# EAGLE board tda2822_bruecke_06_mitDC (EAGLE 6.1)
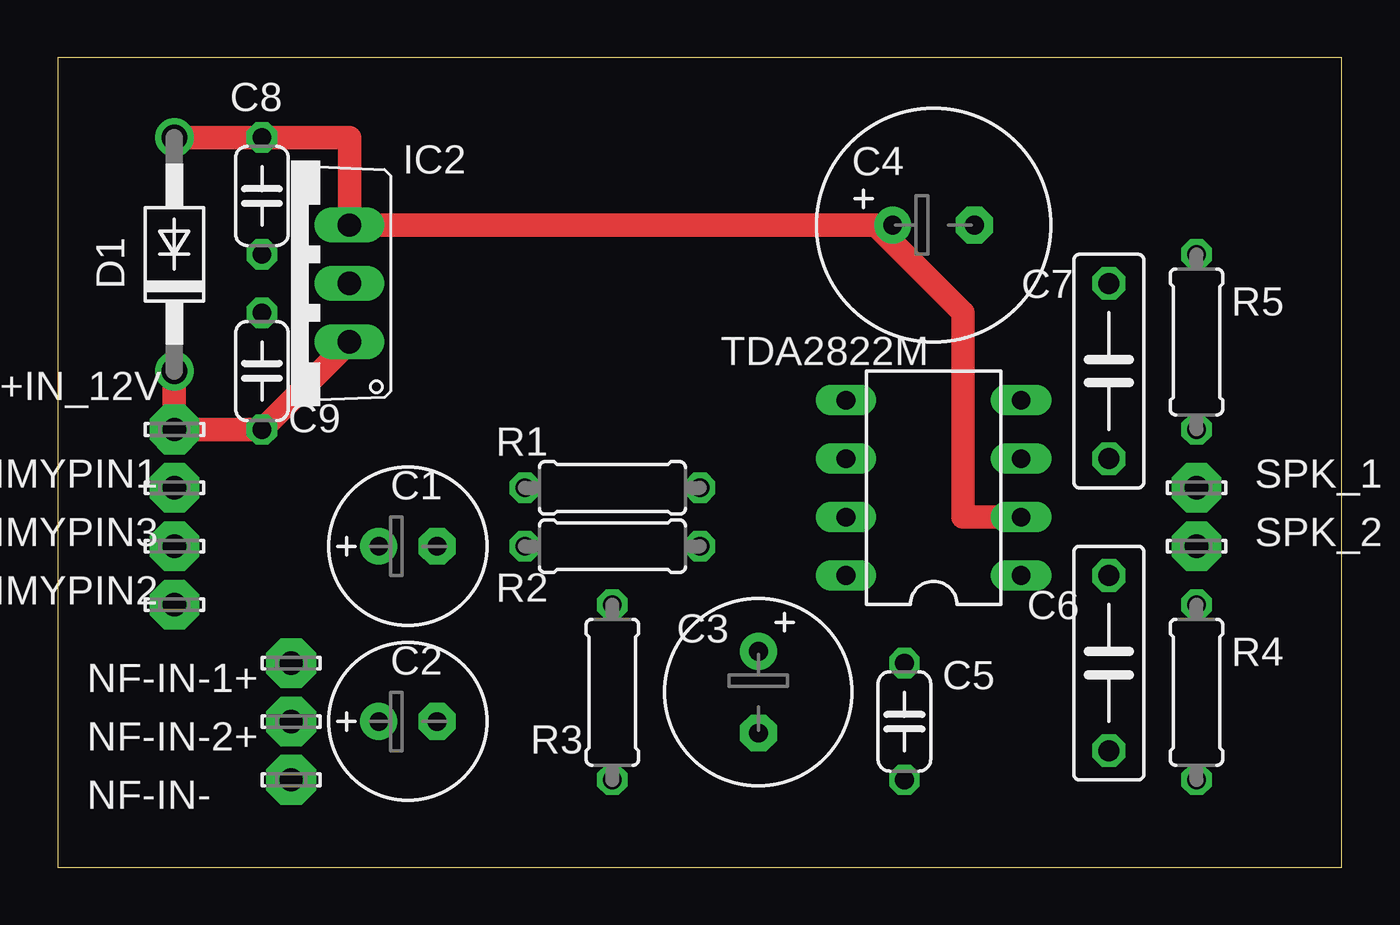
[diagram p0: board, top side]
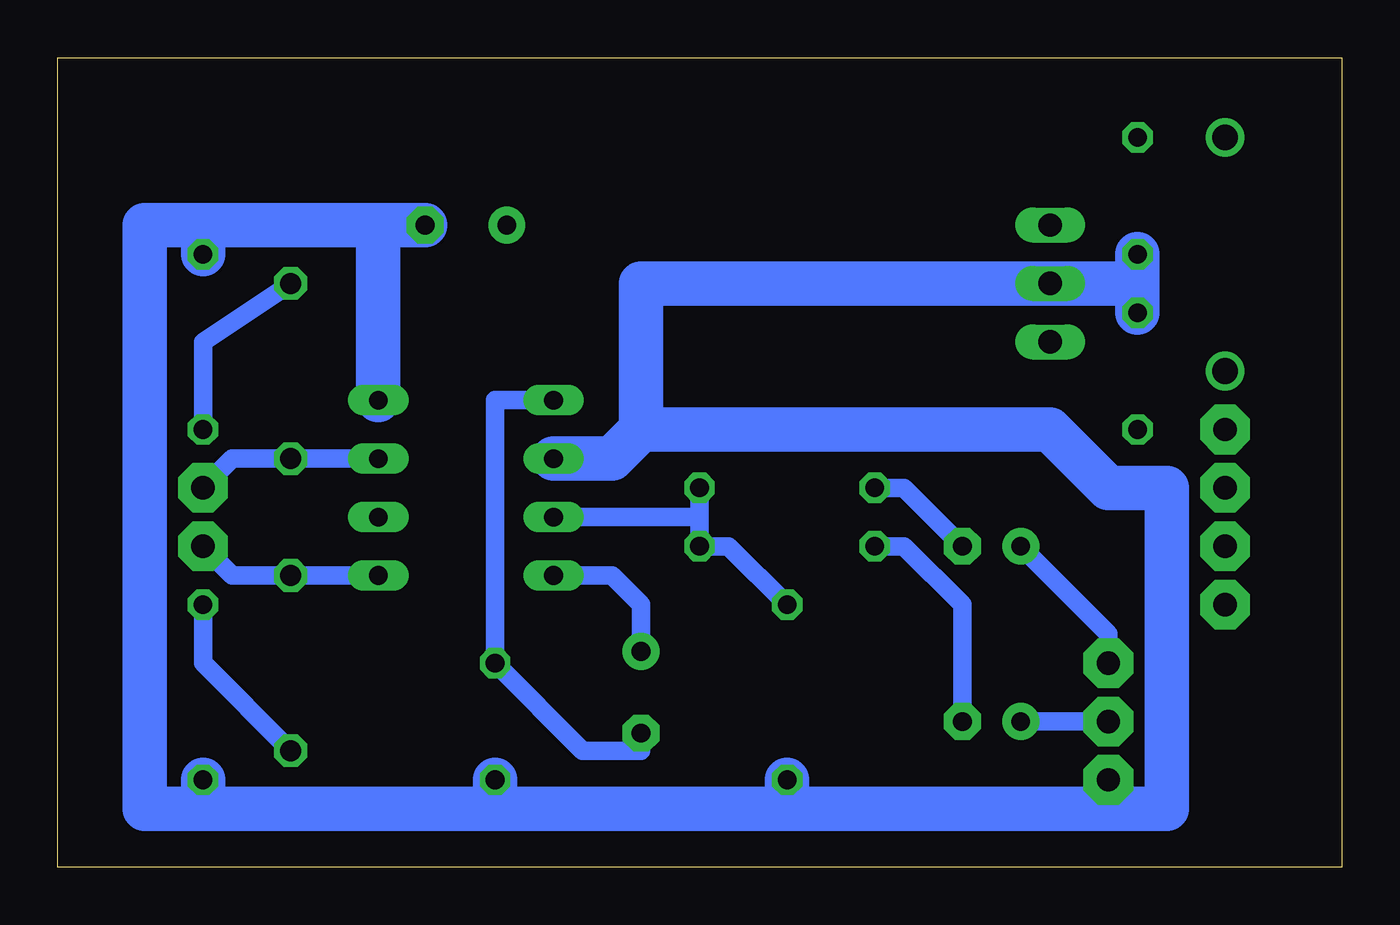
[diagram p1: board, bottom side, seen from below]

Size 55.86 x 35.23 mm. Coordinates in mm from the lower left corner, seen from the top.
Outline: 0,0 55.86,0 55.86,35.23 0,35.23 0,0
Copper layers (1*16): Top 0.035mm / dielectric 1.5mm / Bottom 0.035mm
Design rules: minimum track width 10mil, minimum drill 24mil, track to track 8mil, track to pad 8mil, pad to pad 8mil, via to via 8mil, smd to smd 8mil, copper to edge 40mil, drill to drill 8mil, minimum pad ring 10mil, minimum via ring 8mil, stop-mask expansion 4mil, vias tented up to drill 0mil, thermal gap 10mil

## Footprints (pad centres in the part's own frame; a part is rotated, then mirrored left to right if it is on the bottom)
E2,5-7 = drill 0.813 pad 1.6: + -1.27,0 | drill 0.813 pad 1.6 octagon: - 1.27,0
E3,5-8 = drill 0.813 pad 1.6: + -1.778,0 | drill 0.813 pad 1.6 octagon: - 1.778,0
E3,5-10 = drill 0.813 pad 1.6: + -1.778,0 | drill 0.813 pad 1.6 octagon: - 1.778,0
C050-024X044 = drill 0.813 octagon: 1 -2.54,0; 2 2.54,0
C075-032X103 = drill 0.914 octagon: 1 -3.81,0; 2 3.81,0
DO41-10 = drill 1.118: A 5.08,0; C -5.08,0
LSP10 = drill 1.016 pad 2.159 octagon: MP 0,0
TO220V = drill 1.016 long: 1 -2.54,-2.54; 2 0,-2.54; 3 2.54,-2.54
0207/7 = drill 0.813 octagon: 1 -3.81,0; 2 3.81,0
DIL08 = drill 0.813 long: 1 -3.81,-3.81; 2 -1.27,-3.81; 3 1.27,-3.81; 4 3.81,-3.81; 5 3.81,3.81; 6 1.27,3.81; 7 -1.27,3.81; 8 -3.81,3.81

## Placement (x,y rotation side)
C1  4.7µ  [E2,5-7]  15.24,13.97 0 top
C2  4.7µ  [E2,5-7]  15.24,6.35 0 top
C3  10µ  [E3,5-8]  30.48,7.62 270 top
C4  100µ  [E3,5-10]  38.1,27.94 0 top
C5  10n  [C050-024X044]  36.83,6.35 270 top
C6  100n  [C075-032X103]  45.72,8.89 270 top
C7  100n  [C075-032X103]  45.72,21.59 90 top
C8  330n  [C050-024X044]  8.89,29.21 270 top
C9  330n  [C050-024X044]  8.89,21.59 90 top
D1  1N4004  [DO41-10]  5.08,26.67 90 top
DC+IN_12V  LSP10  [LSP10]  5.08,19.05 0 top
DUMMYPIN1  LSP10  [LSP10]  5.08,16.51 0 top
DUMMYPIN2  LSP10  [LSP10]  5.08,11.43 0 top
DUMMYPIN3  LSP10  [LSP10]  5.08,13.97 0 top
IC2  7806  [TO220V]  10.16,25.4 90 top
NF-IN-  LSP10  [LSP10]  10.16,3.81 0 top
NF-IN-1+  LSP10  [LSP10]  10.16,8.89 0 top
NF-IN-2+  LSP10  [LSP10]  10.16,6.35 0 top
R1  22K  [0207/7]  24.13,16.51 0 top
R2  22K  [0207/7]  24.13,13.97 0 top
R3  2.2K  [0207/7]  24.13,7.62 90 top
R4  10R  [0207/7]  49.53,7.62 90 top
R5  10R  [0207/7]  49.53,22.86 90 top
SPK_1  LSP10  [LSP10]  49.53,16.51 0 top
SPK_2  LSP10  [LSP10]  49.53,13.97 0 top
TDA2822M  [DIL08]  38.1,16.51 90 top

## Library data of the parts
C1-C9 R1-R5 = rcl
D1 = diode
DC+IN_12V DUMMYPIN1-DUMMYPIN3 NF-IN- NF-IN-1+ NF-IN-2+ SPK_1 SPK_2 = solpad
IC2 = linear
TDA2822M = ic-package

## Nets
GND: C4.- C5.2 C8.2 C9.2 IC2.2 NF-IN-.MP R3.1 R4.1 R5.2 TDA2822M.4 TDA2822M.6
N$1: R1.2 R2.2 R3.2 TDA2822M.7
N$2: C5.1 TDA2822M.5
N$3: TDA2822M.8
N$4: C9.1 D1.C DC+IN_12V.MP IC2.1
N$5: C4.+ C8.1 D1.A IC2.3 TDA2822M.2
N$6: C7.1 SPK_1.MP TDA2822M.3
N$7: C7.2 R5.1
N$8: C1.+ NF-IN-1+.MP
N$9: C6.1 SPK_2.MP TDA2822M.1
N$10: C6.2 R4.2
N$11: C2.- R2.1
N$12: C1.- R1.1
N$13: C2.+ NF-IN-2+.MP

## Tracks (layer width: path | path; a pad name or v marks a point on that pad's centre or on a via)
GND
  Bottom 1.93: NF-IN-.MP 10.16,2.54 | 10.16,2.54 7.62,2.54 7.62,16.51 10.16,16.51 12.7,19.05 30.48,19.05 | 10.16,2.54 24.13,2.54 | R3.1 24.13,2.54 | 49.53,27.94 52.07,27.94 52.07,2.54 49.53,2.54 | R5.2 49.53,27.94 | 49.53,27.94 41.91,27.94 | C4.- 41.91,27.94 | 41.91,27.94 TDA2822M.4 | 30.48,19.05 31.75,17.78 TDA2822M.6 | R4.1 49.53,2.54 | 49.53,2.54 36.83,2.54 | 36.83,2.54 C5.2 | 24.13,2.54 36.83,2.54 | C9.2 8.89,25.4 | 8.89,25.4 IC2.2 30.48,25.4 30.48,19.05 | 8.89,25.4 C8.2
N$1
  Bottom 0.813: R3.2 26.67,13.97 R2.2 R1.2 27.94,15.24 TDA2822M.7
N$2
  Bottom 0.813: TDA2822M.5 36.83,20.32 C5.1 33.02,5.08 30.48,5.08 30.48,5.84
N$3
  Bottom 0.813: TDA2822M.8 31.75,12.7 30.48,11.43 30.48,9.4
N$4
  Top 1.016: IC2.1 C9.1 DC+IN_12V.MP D1.C
N$5
  Top 1.016: IC2.3 12.7,30.48 | IC2.3 12.7,31.75 C8.1 D1.A | IC2.3 35.56,27.94 | 35.56,27.94 39.37,24.13 39.37,15.24 TDA2822M.2 | C4.+ 35.56,27.94
N$6
  Bottom 0.813: TDA2822M.3 C7.1 48.26,17.78 SPK_1.MP
N$7
  Bottom 0.813: C7.2 49.53,22.86 R5.1
N$8
  Bottom 0.813: NF-IN-1+.MP 10.16,10.16 C1.+
N$9
  Bottom 0.813: SPK_2.MP 48.26,12.7 C6.1 TDA2822M.1
N$10
  Bottom 0.813: C6.2 49.53,8.89 R4.2
N$11
  Bottom 0.813: C2.- 16.51,11.43 19.05,13.97 R2.1
N$12
  Bottom 0.813: C1.- 19.05,16.51 R1.1
N$13
  Bottom 0.813: NF-IN-2+.MP C2.+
